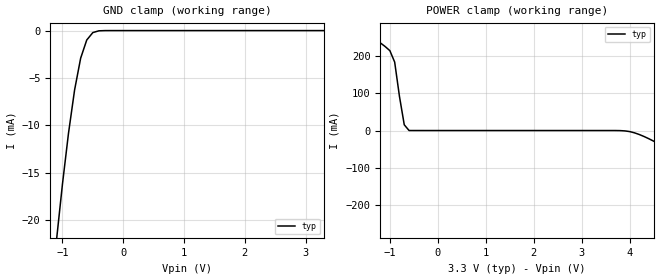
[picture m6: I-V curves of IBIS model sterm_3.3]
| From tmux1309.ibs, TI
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| sterm_3.3
[Model]   sterm_3.3
Model_type   Terminator
|   typ   min   max
C_comp   1.008417e-12   NA   NA
[Voltage Range]   3.3   NA   NA
[Temperature Range]   27   NA   NA
[Power Clamp Reference]   3.3   NA   NA
[GND Clamp Reference]   0   NA   NA
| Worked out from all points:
|   GND clamp passes 1 mA (typ) near -0.60 V on its own axis
|   POWER clamp passes 1 mA (typ) near -0.61 V on its own axis
[GND Clamp]
|   Voltage   I(typ)   I(min)   I(max)
-6.6V     -37.87kA   NA         NA
-1.1V     -22.27mA   NA         NA
-1V       -16.23mA   NA         NA
-900mV    -10.83mA   NA         NA
-800mV    -6.273mA   NA         NA
-700mV    -2.911mA   NA         NA
-600mV    -997uA     NA         NA
-500mV    -212.9uA   NA         NA
-400mV    -24.65uA   NA         NA
-300mV    -1.689uA   NA         NA
3.3V      810.6pA    NA         NA
[POWER Clamp]
|   Voltage   I(typ)   I(min)   I(max)
-3.3V     428.2mA    NA         NA
-1.7V     280.6mA    NA         NA
-1.1V     226.6mA    NA         NA
-900mV    184.5mA    NA         NA
-700mV    15.41mA    NA         NA
-600mV    43.81uA    NA         NA
3.8V      -212.9uA   NA         NA
4.3V      -16.23mA   NA         NA
6.2V      -169.2mA   NA         NA
6.3V      -247.6mA   NA         NA
6.4V      -3.112A    NA         NA
6.6V      -1.138kA   NA         NA
